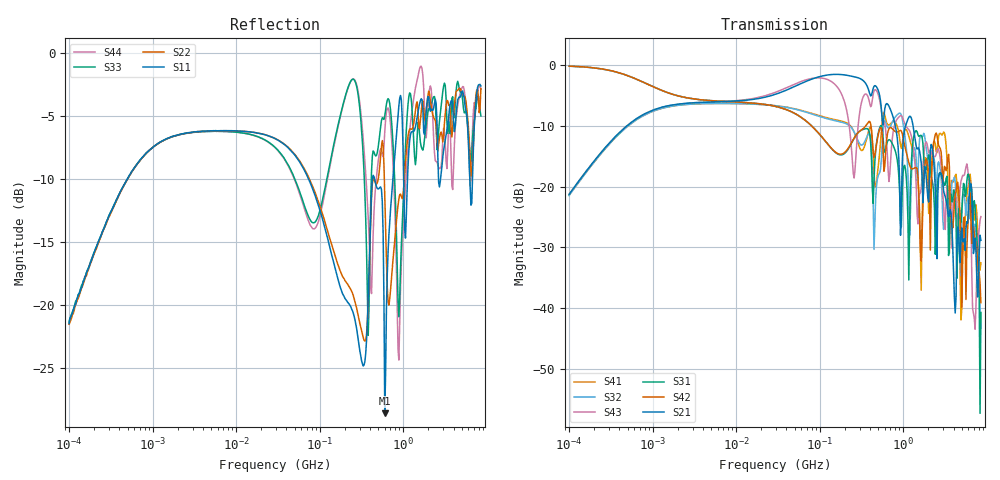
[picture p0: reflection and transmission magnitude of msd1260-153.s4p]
# MHz S MA R 50
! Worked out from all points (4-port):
!   498 points, 100 kHz to 8.5 GHz, reference 50 ohm
!   strongest paths, dB at 100 kHz, 1.698 MHz, 29.49 MHz, 500.7 MHz, 8.5 GHz:
!     S21: -21.3, -6.6, -4.8, -4.1, -28.8
!     S42: -0.2, -4.7, -6.8, -11.5, -39.1
!     S31: -0.2, -4.8, -6.8, -11.3, -40.7
!     S43: -21.2, -6.6, -4.5, -4.8, -24.9
!     S32: -21.5, -6.8, -6.7, -18.2, -43.3
!     S41: -21.4, -6.8, -6.6, -16.8, -32.6
!   lowest |S11| = -28.6 dB at 601 MHz (marker M1), VSWR 1.08, Z = 50.4 - j3.72 ohm
!   |S11| at or under -10 dB: 73.42 MHz to 428.3 MHz (354.9 MHz wide, 141 % of centre); 452.8 MHz to 752.1 MHz (299.3 MHz wide, 49.7 % of centre); 6.258 GHz to 6.749 GHz (491.3 MHz wide, 7.55 % of centre)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
0.1  0.08459 79.8  0.0865 78.6  0.9823 -5.0  0.08499 -101.6
     0.0865 78.6  0.08392 79.2  0.08453 -101.7  0.9816 -5.0
     0.9823 -5.0  0.08453 -101.7  0.08566 79.2  0.08662 78.6
     0.08499 -101.6  0.9816 -5.0  0.08662 78.6  0.08457 79.3
78.73314  0.2996 -51.2  0.7647 -0.1  0.3201 -86.6  0.4033 88.5
          0.7647 -0.1  0.3055 -48.1  0.3988 90.7  0.3199 -86.5
          0.3201 -86.6  0.3988 90.7  0.2147 -10.8  0.7765 -13.8
          0.4033 88.5  0.3199 -86.5  0.7765 -13.8  0.2049 -12.5
601.0223  0.03728 -82.0  0.4371 -97.5  0.1921 -52.5  0.3886 -41.1
          0.4371 -97.5  0.2754 -106.1  0.3478 -17.8  0.148 -28.5
          0.1921 -52.5  0.3478 -17.8  0.5612 -66.3  0.3322 -150.6
          0.3886 -41.1  0.148 -28.5  0.3322 -150.6  0.4862 -52.5
1679.64  0.6494 -155.1  0.1227 118.5  0.257 167.6  0.05258 -87.7
         0.1227 118.5  0.6306 -142.4  0.2558 -168.8  0.04057 -54.1
         0.257 167.6  0.2558 -168.8  0.4148 -149.6  0.118 -138.5
         0.05258 -87.7  0.04057 -54.1  0.118 -138.5  0.8624 -162.7
2972.863  0.3839 99.3  0.1091 -42.1  0.1136 46.7  0.2717 51.6
          0.1091 -42.1  0.4429 91.1  0.05446 8.1  0.1097 33.6
          0.1136 46.7  0.05446 8.1  0.6993 94.6  0.08806 -36.3
          0.2717 51.6  0.1097 33.6  0.08806 -36.3  0.4548 86.8
4588.001  0.6604 -76.8  0.04409 169.9  0.05908 -53.1  0.06974 -164.6
          0.04409 169.9  0.716 -76.3  0.04296 -115.3  0.09545 -144.5
          0.05908 -53.1  0.04296 -115.3  0.7478 -82.1  0.04799 -143.1
          0.06974 -164.6  0.09545 -144.5  0.04799 -143.1  0.6435 -64.6
8500  0.7376 -53.9  0.03626 -92.9  0.009236 -99.4  0.02357 -103.0
      0.03626 -92.9  0.7198 -42.3  0.006837 39.7  0.01109 -124.0
      0.009236 -99.4  0.006837 39.7  0.5612 -48.3  0.05677 -47.4
      0.02357 -103.0  0.01109 -124.0  0.05677 -47.4  0.7163 -54.3
